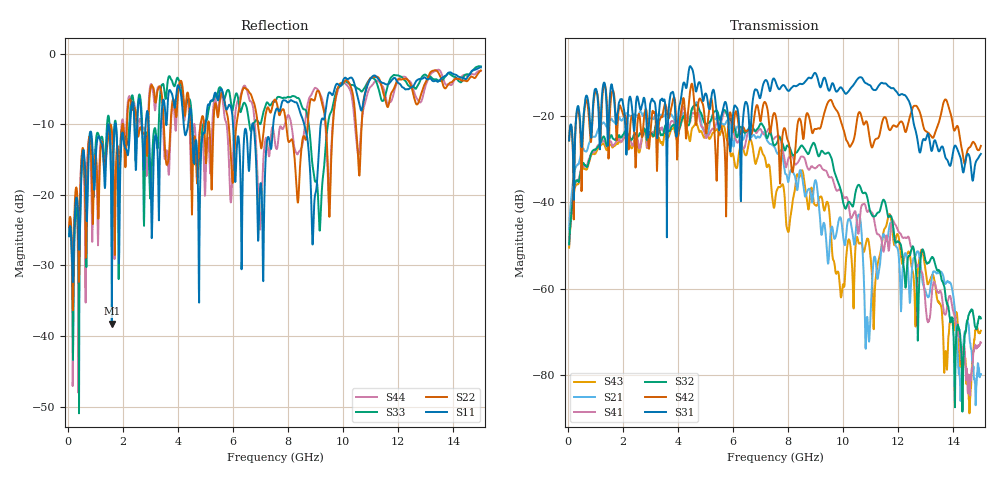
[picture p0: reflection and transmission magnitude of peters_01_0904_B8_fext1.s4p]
# MHZ S RI R 50.00
! FREQ  S11  S12  S13  S14
!  S21  S22  S23  S24
!  S31  S32  S33  S34
!  S41  S42  S43  S44
!  REAL  IMAG  REAL  IMAG  REAL  IMAG  REAL  IMAG
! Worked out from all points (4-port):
!   1496 points, 50 MHz to 15 GHz, reference 50 ohm
!   strongest paths, dB at 50 MHz, 3.79 GHz, 7.53 GHz, 11.27 GHz, 15 GHz:
!     S31: -25.6, -14.5, -11.7, -13.1, -28.8
!     S42: -25.6, -17.2, -19.5, -25.1, -26.9
!     S32: -49.7, -22.3, -26.7, -42.3, -66.9
!     S41: -49.8, -21.1, -24.9, -47.4, -72.6
!     S21: -46.2, -19.9, -27.4, -57.1, -79.8
!     S43: -50.5, -23.0, -39.6, -53.8, -69.8
!   lowest |S11| = -38.2 dB at 1.6 GHz (marker M1), VSWR 1.02, Z = 48.9 + j0.604 ohm
!   |S11| at or under -10 dB: start of sweep to 1.472 GHz; 6.001 GHz to 6.698 GHz (697.7 MHz wide, 11 % of centre); 6.738 GHz to 7.461 GHz (723.1 MHz wide, 10.2 % of centre)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
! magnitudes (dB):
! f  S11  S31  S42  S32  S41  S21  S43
! 50 MHz  -25.9  -25.6  -25.6  -49.7  -49.8  -46.2  -50.5
! 1.6 GHz  -38.2  -12.7  -14.6  -24.5  -26.4  -20.6  -27.0
! 7.31 GHz  -12.0  -13.6  -21.7  -24.0  -22.8  -26.3  -31.3
! 10.58 GHz  -7.0  -11.0  -19.1  -36.0  -46.1  -42.8  -49.6
! 10.87 GHz  -4.6  -12.5  -21.5  -38.7  -42.2  -66.6  -48.4
! 11.74 GHz  -3.8  -13.5  -23.0  -43.2  -45.2  -44.7  -43.9
! 15 GHz  -1.9  -28.8  -26.9  -66.9  -72.6  -79.8  -69.8
